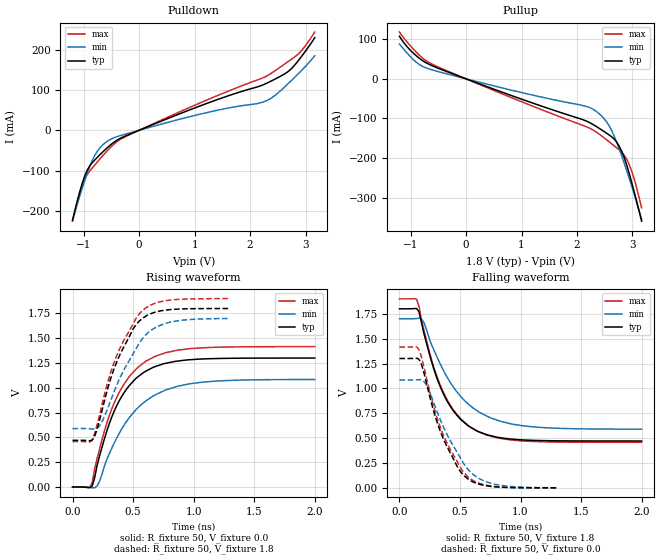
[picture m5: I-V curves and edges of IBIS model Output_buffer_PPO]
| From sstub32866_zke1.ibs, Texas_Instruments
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|   Model   Output_buffer_PPO
[Model]   Output_buffer_PPO
Model_type   Output
Polarity   Non-Inverting
Vmeas  =   0.90
Cref   =   5.00p
Rref   =   1000
Vref   =   0.00
|Variable   typ   min   max
C_comp   1.862e-12   1.304e-12   2.411e-12
|Variable   typ   min   max
[Voltage range]   1.8   1.7   1.9
|Variable   typ   min   max
[Temperature range]  27   125   0.0
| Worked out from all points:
|   slope of the pulldown table from 0 to 0.27 V, typ, clamps not added: 17.6 ohm
|   slope of the pullup table from 0 to 0.27 V, typ, clamps not added: 19.1 ohm
|   rising waveform, R_fixture 50, V_fixture 0.0: 20-80 % time 270ps typ, 340ps min, 280ps max; typ from 0 V to 1.3 V
|   falling waveform, R_fixture 50, V_fixture 1.8: 20-80 % time 264ps typ, 346ps min, 273ps max; typ from 1.8 V to 0.471 V
|   rising waveform, R_fixture 50, V_fixture 1.8: 20-80 % time 240ps typ, 270ps min, 259ps max; typ from 0.471 V to 1.8 V
|   falling waveform, R_fixture 50, V_fixture 0.0: 20-80 % time 232ps typ, 266ps min, 250ps max; typ from 1.3 V to 0 V
[Pulldown]
|Voltage   I(typ)   I(min)   I(max)
-1.2V     -223mA     -222.4mA   -225.7mA
-1.065V   -149.9mA   -160.7mA   -153.3mA
-930mV    -97.39mA   -104.4mA   -108.5mA
-750mV    -66.63mA   -51.22mA   -78.08mA
-570mV    -42.81mA   -26.79mA   -50.13mA
-210mV    -12.01mA   -8.127mA   -13.36mA
1.185V    64.81mA    42.71mA    72.94mA
2.265V    114.5mA    71.51mA    132.1mA
2.445V    126.7mA    86.09mA    147.1mA
2.715V    149.1mA    119.5mA    173.2mA
2.94V     185.5mA    150.3mA    199.5mA
3.165V    229.6mA    184.6mA    243.6mA
[Pullup]
|Voltage   I(typ)   I(min)   I(max)
-1.2V     107.6mA    87.99mA    118.3mA
-1.065V   81.57mA    65.57mA    93.56mA
-885mV    56.96mA    40.67mA    65.76mA
-615mV    33.39mA    22.79mA    37.48mA
2.13V     -104.5mA   -68.3mA    -119mA
2.355V    -121.1mA   -83.08mA   -135.3mA
2.58V     -141.9mA   -118.9mA   -159.3mA
2.715V    -159.9mA   -160.2mA   -174.5mA
2.805V    -183mA     -194.3mA   -185.4mA
2.895V    -217.5mA   -231.3mA   -203.1mA
2.985V    -261.5mA   -270.7mA   -232.9mA
3.165V    -360mA     -355mA     -326mA
[Ramp]
|Variable   typ   min   max
dV/dt_r  0.7803/2.684e-10   0.6509/3.399e-10   0.8494/2.789e-10
dV/dt_f  0.7975/2.628e-10   0.6663/3.456e-10   0.8654/2.709e-10
R_load  =  50
[Rising Waveform]
R_fixture   =   50
V_fixture   =   0.0
V_fixture_min   =   0.0
V_fixture_max   =   0.0
C_fixture   =   0.00
|Time   V(typ)   V(min)   V(max)
0s        646.1nV    1.69uV     0V
141.4ps   -6.95mV    -3.093mV   -4.015mV
161.6ps   8.338mV    -7.282mV   41.19mV
222.2ps   310.6mV    55.58mV    381.6mV
343.4ps   763.6mV    442.2mV    846mV
464.6ps   1.018V     693.2mV    1.109V
606.1ps   1.169V     869.2mV    1.269V
767.7ps   1.247V     978mV      1.354V
1.071ns   1.291V     1.057V     1.403V
2ns       1.3V       1.084V     1.416V
[Falling Waveform]
R_fixture   =   50
V_fixture   =   1.8
V_fixture_min   =   1.7
V_fixture_max   =   1.9
C_fixture   =   0.00
|Time   V(typ)   V(min)   V(max)
0s        1.8V       1.7V       1.9V
141.4ps   1.803V     1.702V     1.897V
161.6ps   1.77V      1.705V     1.824V
202ps     1.552V     1.662V     1.587V
282.8ps   1.199V     1.39V      1.217V
363.6ps   944.2mV    1.18V      958.4mV
505.1ps   688mV      919.9mV    694.3mV
646.5ps   568.2mV    770.7mV    567.4mV
1.051ns   479.9mV    619.4mV    469.1mV
2ns       470.9mV    589.8mV    457.8mV
[Rising Waveform]
R_fixture   =   50
V_fixture   =   1.8
V_fixture_min   =   1.7
V_fixture_max   =   1.9
C_fixture   =   0.00
|Time   V(typ)   V(min)   V(max)
0s        470.8mV    589.4mV    457.7mV
144.4ps   466.8mV    587.2mV    455.4mV
170.7ps   485.2mV    584.4mV    495.2mV
236.4ps   737.8mV    643.2mV    794.4mV
354.5ps   1.23V      996.2mV    1.294V
499ps     1.591V     1.339V     1.643V
577.8ps   1.701V     1.497V     1.78V
696ps     1.767V     1.616V     1.859V
814.1ps   1.789V     1.665V     1.886V
1.3ns     1.8V       1.699V     1.9V
[Falling Waveform]
R_fixture   =   50
V_fixture   =   0.0
V_fixture_min   =   0.0
V_fixture_max   =   0.0
C_fixture   =   0.00
|Time   V(typ)   V(min)   V(max)
0s        1.3V       1.085V     1.416V
157.6ps   1.295V     1.087V     1.397V
183.8ps   1.234V     1.084V     1.306V
223.2ps   1.057V     1.032V     1.106V
275.8ps   801.8mV    880.6mV    845.4mV
341.4ps   556.2mV    672.6mV    596.3mV
472.7ps   224.8mV    365.7mV    273.7mV
564.6ps   90.29mV    188.6mV    111.4mV
787.9ps   10.47mV    35.49mV    13.53mV
1.3ns     59.91uV    776.1uV    89.27uV
